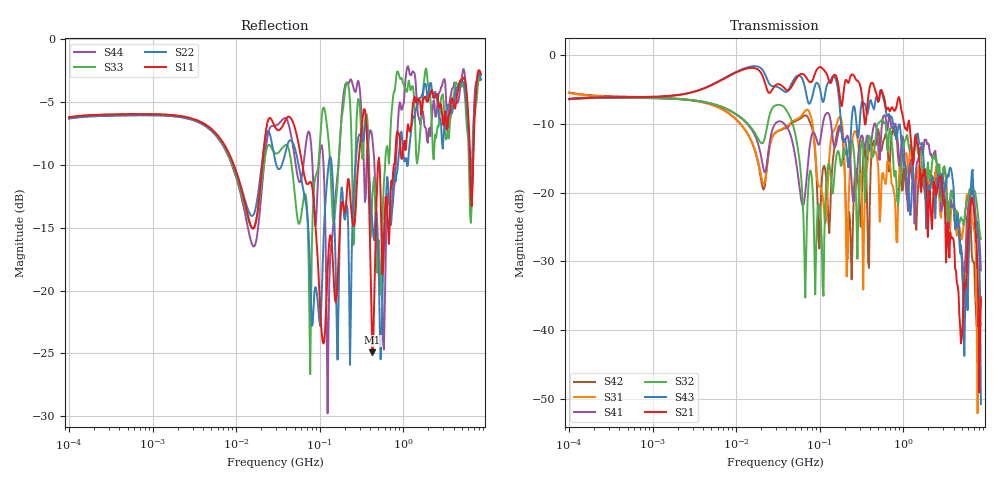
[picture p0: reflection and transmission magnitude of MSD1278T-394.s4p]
# MHz S MA R 50
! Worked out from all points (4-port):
!   498 points, 100 kHz to 8.5 GHz, reference 50 ohm
!   strongest paths, dB at 100 kHz, 1.698 MHz, 29.49 MHz, 500.7 MHz, 8.5 GHz:
!     S21: -6.4, -5.9, -4.4, -6.8, -35.2
!     S43: -6.4, -5.9, -4.6, -6.9, -50.8
!     S32: -6.4, -6.4, -7.3, -10.0, -26.7
!     S41: -6.4, -6.4, -10.0, -13.1, -31.3
!     S31: -5.5, -6.4, -11.3, -16.2, -39.1
!     S42: -5.5, -6.3, -11.3, -10.8, -35.7
!   lowest |S11| = -24.9 dB at 426.7 MHz (marker M1), VSWR 1.12, Z = 45.3 + j2.76 ohm
!   |S11| at or under -10 dB: 62.01 MHz to 288.9 MHz (226.9 MHz wide, 129 % of centre); 520.3 MHz to 771.7 MHz (251.4 MHz wide, 38.9 % of centre); 6.332 GHz to 6.852 GHz (520.1 MHz wide, 7.89 % of centre)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
0.1  0.4893 12.0  0.4777 13.2  0.5288 -12.3  0.4762 -168.1
     0.4777 13.2  0.4834 12.0  0.4761 -168.0  0.5328 -12.2
     0.5288 -12.3  0.4761 -168.0  0.4878 12.0  0.4794 13.1
     0.4762 -168.1  0.5328 -12.2  0.4794 13.1  0.4823 12.3
426.6928  0.05671 147.6  0.6273 -65.8  0.2039 -42.6  0.2685 -3.4
          0.6273 -65.8  0.1857 -85.8  0.1802 -13.4  0.2147 22.3
          0.2039 -42.6  0.1802 -13.4  0.2372 -53.0  0.4299 -60.2
          0.2685 -3.4  0.2147 22.3  0.4299 -60.2  0.4035 -88.9
1113.489  0.4298 -95.9  0.2815 -162.2  0.1786 -111.8  0.09411 -150.3
          0.2815 -162.2  0.3127 -103.9  0.2624 -106.9  0.09145 -130.5
          0.1786 -111.8  0.2624 -106.9  0.617 -122.3  0.1172 161.2
          0.09411 -150.3  0.09145 -130.5  0.1172 161.2  0.7716 -102.3
2972.863  0.4663 84.6  0.08859 -62.4  0.1352 77.9  0.09133 54.3
          0.08859 -62.4  0.3666 90.5  0.1368 72.9  0.0805 50.0
          0.1352 77.9  0.1368 72.9  0.6034 78.0  0.1304 -16.8
          0.09133 54.3  0.0805 50.0  0.1304 -16.8  0.6729 95.2
5142.985  0.6947 -100.0  0.01082 -167.2  0.0502 -119.6  0.03042 -138.7
          0.01082 -167.2  0.6784 -100.1  0.06352 -116.8  0.02401 -166.2
          0.0502 -119.6  0.06352 -116.8  0.6579 -103.0  0.02278 -40.7
          0.03042 -138.7  0.02401 -166.2  0.02278 -40.7  0.7404 -96.4
6764.496  0.2707 59.4  0.08701 12.4  0.05915 30.4  0.09789 72.7
          0.08701 12.4  0.2818 66.9  0.112 68.0  0.03175 26.1
          0.05915 30.4  0.112 68.0  0.3316 56.1  0.1463 35.1
          0.09789 72.7  0.03175 26.1  0.1463 35.1  0.3684 67.2
8500  0.725 -55.6  0.01733 -21.8  0.01113 -34.0  0.02724 -149.9
      0.01733 -21.8  0.6913 -59.3  0.04601 -142.4  0.01638 -42.1
      0.01113 -34.0  0.04601 -142.4  0.7208 -45.7  0.0029 -1.4
      0.02724 -149.9  0.01638 -42.1  0.0029 -1.4  0.692 -49.8
